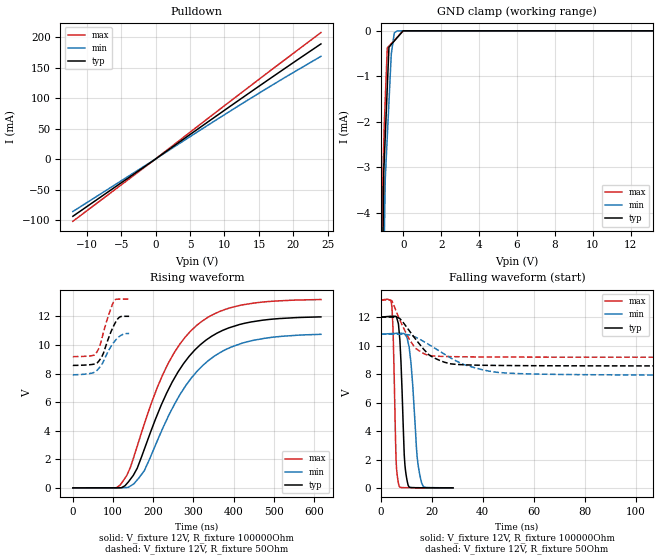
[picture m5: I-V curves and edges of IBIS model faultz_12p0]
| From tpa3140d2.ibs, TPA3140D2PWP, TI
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|   faultz_12p0 Model
[Model]   faultz_12p0
Model_type   Open_drain
Polarity   Non-Inverting
Vmeas = 6
Vref = 12
Cref = 2pF
Rref = 100000
|   typ   min   max
|   (nom PVT)   (fast PVT)   (slow PVT)
C_comp   1.649e-13   1.526e-13   1.894e-13
| Where nom  PVT is Nominal Process, 12V, 27C
|   Fast PVT is Strong Process,  13.2V, -40C
|   Slow PVT is Weak Process,   10.8V, 125C
[Voltage Range]   12   10.8   13.2
|Junction Temperature
[Temperature Range]   27   125   -40
[Pullup Reference]   12   10.8   13.2
[Pulldown Reference]   0   0   0
[Power Clamp Reference]   12   10.8   13.2
[GND Clamp Reference]   0   0   0
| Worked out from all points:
|   slope of the pulldown table from 0 to 1.8 V, typ, clamps not added: 124 ohm
|   GND clamp passes 1 mA (typ) near -0.82 V on its own axis
|   falling waveform, V_fixture 12V, R_fixture 100000Ohm: 20-80 % time 1.47ns typ, 2.37ns min, 1.01ns max; typ from 12 V to 0.019 V
|   rising waveform, V_fixture 12V, R_fixture 100000Ohm: 20-80 % time 127ns typ, 132ns min, 122ns max; typ from 0.015 V to 12 V
|   falling waveform, V_fixture 12V, R_fixture 50Ohm: 20-80 % time 9.67ns typ, 18.3ns min, 6.83ns max; typ from 12 V to 8.57 V
|   rising waveform, V_fixture 12V, R_fixture 50Ohm: 20-80 % time 27.8ns typ, 35ns min, 25.1ns max; typ from 8.57 V to 12 V
[Pulldown]
|   Voltage   I(typ)   I(min)   I(max)
-12V      -93.86mA   -86.07mA   -102.1mA
0V        0A         0A         0A
11.99V    95.69mA    86.87mA    104.7mA
24V       188.8mA    168.5mA    207.4mA
[GND Clamp]
|   Voltage   I(typ)   I(min)   I(max)
-12V      -702.1mA   -501.3mA   -935.5mA
-1.188V   -9.159mA   -10.48mA   -6.662mA
-1.109V   -6.096mA   -7.732mA   -4.009mA
-1.058V   -4.148mA   -5.984mA   -2.954mA
-1.032V   -3.127mA   -5.315mA   -2.491mA
-1.003V   -2.838mA   -4.586mA   -2.063mA
-950.4mV  -2.309mA   -3.247mA   -1.501mA
-844.8mV  -1.25mA    -2.335mA   -375.9uA
-756mV    -359.3uA   -1.568mA   -336.3uA
-626.4mV  -296.7uA   -487.7uA   -278.7uA
-324mV    -150.7uA   -1.501uA   -144.1uA
24V       0A         0A         0A
[POWER Clamp]
|   Voltage   I(typ)   I(min)   I(max)
-12V      0A         0A         0A
0V        0A         0A         0A
24V       0A         0A         0A
[Ramp]
R_load = 100000
|   typ   min   max
dV/dt_r   7.18276/1.27764e-07   6.4588/1.32629e-07   7.90541/1.22797e-07
dV/dt_f   7.19102/1.4724e-09   6.47097/2.3749e-09   7.91095/1.01267e-09
[Falling Waveform]
V_fixture = 12V
V_fixture_min = 10.8V
V_fixture_max = 13.2V
R_fixture = 100000Ohm
|   Time   V(typ)   V(min)   V(max)
0s        12V        10.8V      13.2V
4.48ns    12.06V     10.85V     12.68V
5.024ns   12.06V     10.85V     10.29V
6.072ns   12.04V     10.86V     2.072V
7.196ns   11.16V     10.87V     187.9mV
9.286ns   2.356V     10.83V     33.14mV
10.86ns   185.5mV    10.18V     27.91mV
14.33ns   30.22mV    2.224V     24.09mV
16.12ns   25.05mV    359.8mV    22.46mV
28.4ns    18.99mV    23.57mV    18.91mV
[Rising Waveform]
V_fixture = 12V
V_fixture_min = 10.8V
V_fixture_max = 13.2V
R_fixture = 100000Ohm
|   Time   V(typ)   V(min)   V(max)
0s        14.9mV     14.63mV    15mV
117.8ns   21.24mV    17.91mV    218.5mV
150.3ns   883.9mV    268.1mV    2.06V
178ns     2.726V     1.224V     4.498V
238.5ns   6.923V     5.072V     8.777V
275.4ns   8.696V     6.922V     10.4V
322.5ns   10.14V     8.545V     11.68V
379.2ns   11.09V     9.663V     12.48V
435.2ns   11.56V     10.23V     12.86V
617.2ns   11.96V     10.74V     13.17V
[Falling Waveform]
V_fixture = 12V
V_fixture_min = 10.8V
V_fixture_max = 13.2V
R_fixture = 50Ohm
|   Time   V(typ)   V(min)   V(max)
0s        12V        10.8V      13.2V
4.531ns   12V        10.8V      13.12V
7.572ns   11.9V      10.8V      11.8V
11.33ns   11.03V     10.75V     10.43V
13.57ns   10.49V     10.6V      9.833V
18.9ns    9.368V     10.08V     9.314V
25.05ns   8.834V     9.402V     9.239V
32.56ns   8.657V     8.676V     9.215V
45.73ns   8.609V     8.125V     9.201V
139.8ns   8.575V     7.927V     9.186V
[Rising Waveform]
V_fixture = 12V
V_fixture_min = 10.8V
V_fixture_max = 13.2V
R_fixture = 50Ohm
|   Time   V(typ)   V(min)   V(max)
0s        8.572V     7.914V     9.185V
45.48ns   8.627V     8.021V     9.241V
57.48ns   8.7V       8.151V     9.405V
65.43ns   8.902V     8.396V     9.789V
72.35ns   9.193V     8.661V     10.47V
86.65ns   10.31V     9.481V     11.89V
102.7ns   11.4V      10.21V     13.09V
115.8ns   11.94V     10.59V     13.2V
128ns     12V        10.77V     13.2V
140ns     12V        10.8V      13.2V
